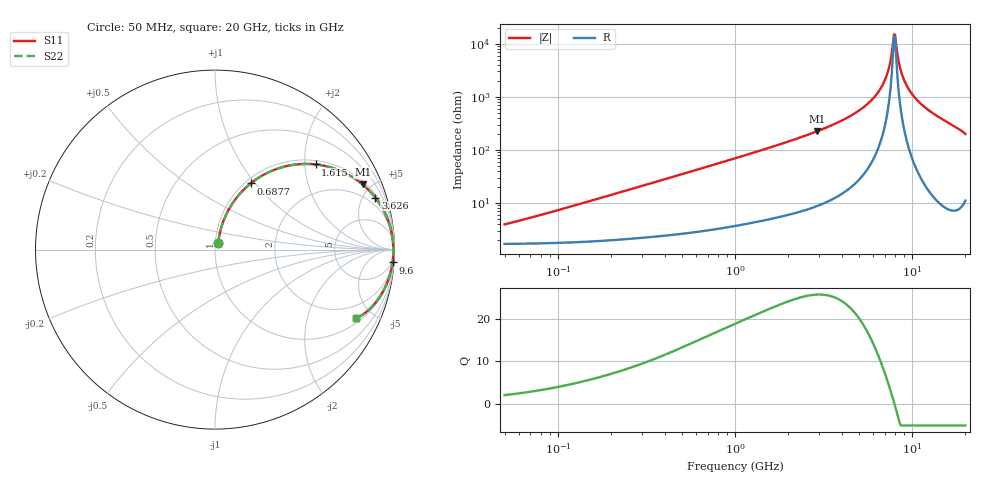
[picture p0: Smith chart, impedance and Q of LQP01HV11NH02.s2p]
!Murata Part Number: LQP01HV11NH02
!These Parameters are Measured in Series Mode Connection
!  o--[Z]--o
!Port1  Port2
!  o-------o
!Freq. Start=50[MHz] Stop=20[GHz], 401[Steps]
# Hz S RI R 50
!Freq.(Hz) S11(Real) S11(Imag) S21(Real) S21(Imag) S12(Real) S12(Imag) S22(Real) S22(Imag)
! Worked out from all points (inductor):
!   401 points, 50 MHz to 20 GHz, reference 50 ohm
!   read as one part in series: L = 11.3 nH near 72.71 MHz
!   highest Q = 25.7 at 2.896 GHz (marker M1), where L = 12.2 nH
!   self-resonance near 7.902 GHz
!   S11 on the Smith chart (normalised r, x): 50 MHz: 1.03, +0.07; 687.7 MHz: 1.06, +0.95; 1.615 GHz: 1.10, +2.27; 3.626 GHz: 1.24, +6.08; 9.6 GHz: 3, -27; 20 GHz: 1.22, -3.98
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5e7  0.0178 0.0343  0.9822 -0.0343  0.9822 -0.0343  0.0178 0.0343
1.364002e8  0.0267 0.092  0.9733 -0.092  0.9733 -0.092  0.0267 0.092
3.721004e8  0.0814 0.2318  0.9186 -0.2318  0.9186 -0.2318  0.0814 0.2318
6.87656e8  0.1989 0.3688  0.8011 -0.3688  0.8011 -0.3688  0.1989 0.3688
1e9  0.3318 0.445  0.6682 -0.445  0.6682 -0.445  0.3318 0.445
1.614971e9  0.5604 0.4747  0.4396 -0.4747  0.4396 -0.4747  0.5604 0.4747
2.728004e9  0.8007 0.3804  0.1993 -0.3804  0.1993 -0.3804  0.8007 0.3804
2.896447e9  0.8229 0.3628  0.1771 -0.3628  0.1771 -0.3628  0.8229 0.3628
3.626126e9  0.8933 0.2895  0.1067 -0.2895  0.1067 -0.2895  0.8933 0.2895
4.81993e9  0.9539 0.1873  0.0461 -0.1873  0.0461 -0.1873  0.9539 0.1873
5.944466e9  0.9802 0.1095  0.0198 -0.1095  0.0198 -0.1095  0.9802 0.1095
6.802353e9  0.9897 0.059  0.0103 -0.059  0.0103 -0.059  0.9897 0.059
7.114996e9  0.9917 0.0422  0.00832 -0.0422  0.00832 -0.0422  0.9917 0.0422
7.442007e9  0.993 0.0253  0.00697 -0.0253  0.00697 -0.0253  0.993 0.0253
7.784049e9  0.9938 0.00833  0.00621 -0.00833  0.00621 -0.00833  0.9938 0.00833
8.020766e9  0.994 -0.00299  0.00603 0.00299  0.00603 0.00299  0.994 -0.00299
8.141811e9  0.994 -0.00866  0.00605 0.00866  0.00605 0.00866  0.994 -0.00866
8.774992e9  0.9929 -0.0371  0.00712 0.0371  0.00712 0.0371  0.9929 -0.0371
9.600142e9  0.9893 -0.0715  0.0107 0.0715  0.0107 0.0715  0.9893 -0.0715
1.066139e10  0.9818 -0.1121  0.0182 0.1121  0.0182 0.1121  0.9818 -0.1121
1.238412e10  0.9641 -0.1713  0.0359 0.1713  0.0359 0.1713  0.9641 -0.1713
2e10  0.7865 -0.383  0.2135 0.383  0.2135 0.383  0.7865 -0.383
